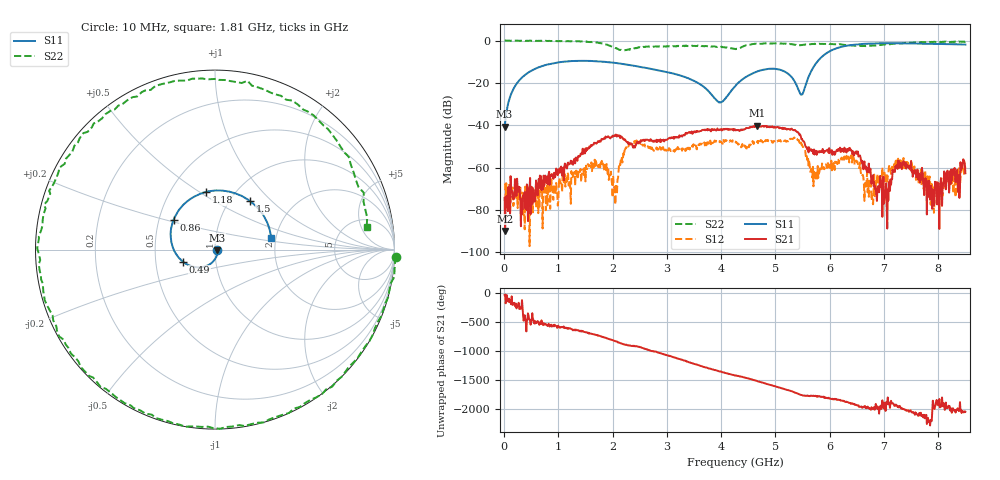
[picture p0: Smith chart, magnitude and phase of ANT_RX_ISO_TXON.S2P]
!Agilent Technologies,E5071C,MY46523237,B.13.01
!Date: Tue Sep 12 16:52:18 2023
!Data & Calibration Information:
!Freq	S11:SOLT2(ON)	S21:SOLT2(ON)	S12:SOLT2(ON)	S22:SOLT2(ON)
!PortZ  Port1:50+j0  Port2:50+j0
!Above PortZ is port z conversion or system Z0 setting when saving the data.
!When reading, reference impedance value at option line is always used.
# Hz S dB R 50
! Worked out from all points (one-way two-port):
!   850 points, 10 MHz to 8.5 GHz, reference 50 ohm
!   highest |S21| = -40.22 dB at 4.66 GHz (marker M1); lowest = -89.9 dB at 20 MHz (marker M2)
!   lowest |S11| = -40.6 dB at 10 MHz (marker M3), VSWR 1.02, Z = 50.9 - j0.173 ohm
!   |S11| at or under -10 dB: start of sweep to 1.081 GHz; 1.85 GHz to 5.769 GHz (3.92 GHz wide, 103 % of centre)
!   |S22| runs from -4.6 to 0.1 dB; largest |S21 - S12| = 0.0093
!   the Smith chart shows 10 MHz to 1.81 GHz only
!   S11 on the Smith chart (normalised r, x): 10 MHz: 1.02, -0.00; 490 MHz: 0.69, -0.10; 860 MHz: 0.60, +0.22; 1.18 GHz: 0.74, +0.53; 1.5 GHz: 1.23, +0.75; 1.81 GHz: 1.89, +0.26
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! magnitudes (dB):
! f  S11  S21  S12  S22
! 10 MHz  -40.6  -74.2  -67.4  0.1
! 20 MHz  -38.8  -89.9  -67.6  0.0
! 490 MHz  -14.4  -81.9  -69.2  0.0
! 860 MHz  -10.9  -63.3  -68.8  -0.2
! 1.18 GHz  -9.8  -57.6  -63.2  -0.2
! 1.43 GHz  -9.5  -53.7  -63.3  -0.4
! 1.5 GHz  -9.5  -50.9  -66.5  -0.5
! 1.81 GHz  -9.9  -46.7  -58.4  -1.4
! 2.04 GHz  -10.5  -44.7  -70.7  -3.3
! 2.28 GHz  -11.4  -47.8  -49.8  -4.2
! 2.84 GHz  -14.1  -46.9  -51.4  -2.8
! 3.97 GHz  -29.0  -42.0  -48.0  -3.0
! 4.26 GHz  -21.4  -42.0  -47.6  -3.9
! 4.66 GHz  -14.6  -40.2  -47.9  -1.5
! 5.39 GHz  -21.1  -42.8  -46.3  -2.1
! 5.67 GHz  -13.9  -52.2  -61.7  -1.6
! 6.5 GHz  -1.8  -52.3  -57.2  -2.4
! 6.76 GHz  -1.4  -64.1  -67.8  -2.4
! 7.09 GHz  -1.2  -66.8  -59.7  -1.6
! 7.27 GHz  -1.3  -59.6  -57.1  -1.5
! 7.89 GHz  -1.5  -79.5  -68.9  -0.7
! 8.5 GHz  -1.9  -62.6  -60.4  -0.5
